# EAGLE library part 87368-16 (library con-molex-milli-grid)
RECEPTACAL
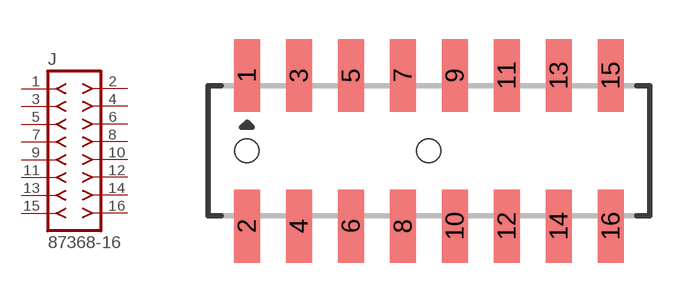
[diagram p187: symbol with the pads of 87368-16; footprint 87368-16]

Designator prefix J

## 87368-16  [87368-16]
1  1  pas
2  2  pas
3  3  pas
4  4  pas
5  5  pas
6  6  pas
7  7  pas
8  8  pas
9  9  pas
10  10  pas
11  11  pas
12  12  pas
13  13  pas
14  14  pas
15  15  pas
16  16  pas

## Footprint 87368-16 (pad centres in mm)
RECEPTACAL SMD Dual Row, Side Entry
smd 1 x 2.8: 1 -7,2.9; 2 -7,-2.9; 3 -5,2.9; 4 -5,-2.9; 5 -3,2.9; 6 -3,-2.9; 7 -1,2.9; 8 -1,-2.9; 9 1,2.9; 10 1,-2.9; 11 3,2.9; 12 3,-2.9; 13 5,2.9; 14 5,-2.9; 15 7,2.9; 16 7,-2.9
hole 0.914 at -7,0
hole 0.914 at 0,0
